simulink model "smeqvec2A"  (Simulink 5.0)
settings: Solver=ode45  StartTime=0.0  StopTime=3  MaxStep=1e-3  RelTol=1e-4  AbsTol=1e-4
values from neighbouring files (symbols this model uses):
  Bm = 0.10    (= 0.1)    [IMabc2.m]    (also in imabcparam.m = 0.01; IMabcrun0.m = 0.01; IMabcrun1.m = 0.001; IMcur0.m = 1e-06)
  H = 0.60    (= 0.6)    [IMabc2.m]    (also in IMcur0.m = 0.3; imdef0vec.m = 0.3; imdef1vec.m = 0.3; imdef2vec.m = 0.3)
  n0 = 0.98    [imdef0vec.m]    (also in imdef1vec.m = 0.978; imdef2vec.m; imdefrotflux.m; imdefSIvec1.m = 0.95)
  Te0 = 0.75/wo*p*(Is*conj(Is)*Req)    [imdefSIvec1.m]
  V = [Vas 0 0].'    [Actac.m]    (also in acttrcalc1.m = str2num(get(h,'string')); im3d.m = eval(get(hVs,'String')); IMabc2.m = [vas vbs vcs 0 0 0]'; IMabcf0.m = [vas vbs vcs 0 0 0]')
  wo = 2*pi*freq0    [calc0.m]    (also in IMabc2.m = 376.991118431; imabcparam.m = 376.991118431; IMabcrun0.m = 376.991118431; IMabcrun1.m = 376.991118431)
undefined symbols (not defined in the file or in its folder): delta0, fk0, L_1, ph, phif0, Rf, Rkd, Rkq, vf0
libraries: simulink x1

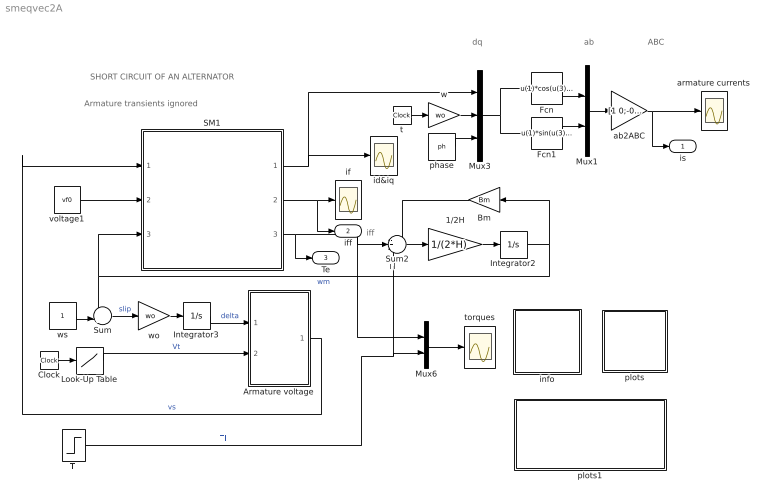
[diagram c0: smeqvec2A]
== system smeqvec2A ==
  note: Tl
  note: SHORT CIRCUIT OF AN ALTERNATOR
  note: iff
  note: Armature transients ignored
  note: ab
  note: ABC
  note: dq
  1/2H : Gain  Gain=1/(2*H)
  Armature voltage : Subsystem
  Bm : Gain  Orientation=left  Gain=Bm
  Clock : Clock
  Fcn : Fcn  Expr=u(1)*cos(u(3)+u(4))-u(2)*sin(u(3)+u(4))
  Fcn1 : Fcn  Expr=u(1)*sin(u(3)+u(4))+u(2)*cos(u(3)+u(4))
  Integrator2 : Integrator  InitialCondition=n0
  Integrator3 : Integrator  InitialCondition=delta0
  Look-Up Table : Lookup  InputValues=[0 0.1 0.1 5]  OutputValues=[V V 0 0]
  Mux1 : Mux  Inputs=2
  Mux3 : Mux  Inputs=3
  Mux6 : Mux  Inputs=2
  SM1 : Subsystem
  Sum : Sum  Inputs=-+|
  Sum2 : Sum  Inputs=-+-
  Tl : Step  Time=0  After=Te0  SampleTime=0
  ab2ABC : Gain  Gain=[1 0;-0.5 sqrt(3)/2;-0.5 -sqrt(3)/2]  Multiplication=Matrix(K*u)
  armature currents : Scope
  id&iq : Scope
  if : Scope
  info : Subsystem
  phase : Constant  Value=ph
  plots : Subsystem
  plots1 : Subsystem
  t : Clock
  torques : Scope
  voltage1 : Constant  Value=vf0
  w : Gain  Gain=wo
  wo : Gain  Gain=wo
  ws : Constant
  is : Outport
  iff : Outport  Port=2
  Te : Outport  Port=3
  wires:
  voltage1/1 -> SM1/2(vf)
  1/2H/1 -> Integrator2/1
  Sum2/1 -> 1/2H/1
  Bm/1 -> Sum2/1
  Mux6/1 -> torques/1
  ws/1 -> Sum/2
  Sum/1 -> wo/1  "slip"
  Armature voltage/1(vs) -> SM1/1(vs)  "vs"
  wo/1 -> Integrator3/1
  Integrator3/1 -> Armature voltage/1(delta)  "delta"
  Clock/1 -> Look-Up Table/1
  Look-Up Table/1 -> Armature voltage/2(Vt)  "Vt"
  Integrator2/1 -> Bm/1, Sum/1, SM1/3(wm)  "wm"
  Tl/1 -> Mux6/2, Sum2/3  "Tl"
  w/1 -> Mux3/2
  phase/1 -> Mux3/3
  t/1 -> w/1
  SM1/2(if) -> if/1, iff/1
  SM1/1(ia) -> id&iq/1, Mux3/1
  SM1/3(Te) -> Sum2/2, Mux6/1, Te/1
  Mux3/1 -> Fcn/1, Fcn1/1
  Fcn1/1 -> Mux1/2
  Fcn/1 -> Mux1/1
  Mux1/1 -> ab2ABC/1
  ab2ABC/1 -> armature currents/1, is/1

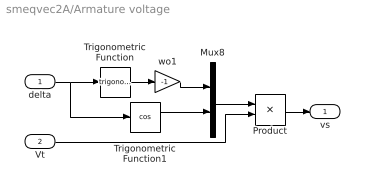
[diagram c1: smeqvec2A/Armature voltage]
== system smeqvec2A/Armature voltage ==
  delta : Inport
  Vt : Inport  Port=2
  Mux8 : Mux  Inputs=2
  Product : Product
  Trigonometric Function : Trigonometry
  Trigonometric Function1 : Trigonometry  Operator=cos
  wo1 : Gain  Gain=-1
  vs : Outport
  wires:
  delta/1 -> Trigonometric Function/1, Trigonometric Function1/1
  Trigonometric Function/1 -> wo1/1
  Mux8/1 -> Product/1
  wo1/1 -> Mux8/1
  Trigonometric Function1/1 -> Mux8/2
  Product/1 -> vs/1
  Vt/1 -> Product/2

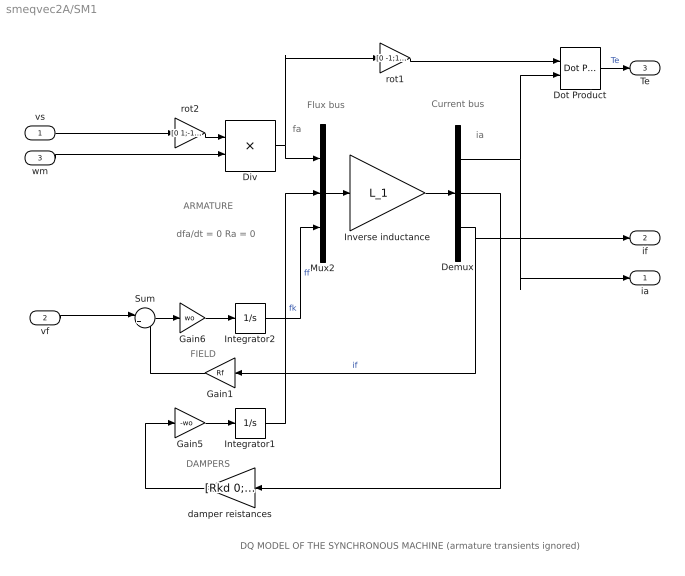
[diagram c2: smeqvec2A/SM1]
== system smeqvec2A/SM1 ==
  note: DAMPERS
  note: ARMATURE
  note: fa
  note: ia
  note: FIELD
  note: DQ MODEL OF THE SYNCHRONOUS MACHINE (armature transients ignored)
  note: Flux bus
  note: Current bus
  note: dfa/dt = 0 Ra = 0
  vs : Inport
  vf : Inport  Port=2
  wm : Inport  Port=3
  Demux : Demux  Outputs=3
  Div : Product  Inputs=*/  Multiplication=Matrix(*)
  Dot Product : simulink/Math Operations/Dot Product
  Gain1 : Gain  Orientation=left  Gain=Rf
  Gain5 : Gain  Gain=-wo
  Gain6 : Gain  Gain=wo
  Integrator1 : Integrator  InitialCondition=fk0
  Integrator2 : Integrator  InitialCondition=phif0
  Inverse inductance : Gain  Gain=L_1  Multiplication=Matrix(K*u)
  Mux2 : Mux  Inputs=3
  Sum : Sum  Inputs=|+-
  damper reistances : Gain  Orientation=left  Gain=[Rkd 0;0 Rkq]  Multiplication=Matrix(K*u)
  rot1 : Gain  Gain=[0 -1;1 0]  Multiplication=Matrix(K*u)
  rot2 : Gain  Gain=[0 1;-1 0]  Multiplication=Matrix(K*u)
  ia : Outport
  if : Outport  Port=2
  Te : Outport  Port=3
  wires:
  Gain5/1 -> Integrator1/1
  damper reistances/1 -> Gain5/1
  vs/1 -> rot2/1
  Gain6/1 -> Integrator2/1
  Sum/1 -> Gain6/1
  vf/1 -> Sum/1
  Gain1/1 -> Sum/2
  rot1/1 -> Dot Product/1
  Demux/1 -> Dot Product/2, ia/1
  Dot Product/1 -> Te/1  "Te"
  Mux2/1 -> Inverse inductance/1
  Inverse inductance/1 -> Demux/1
  Integrator1/1 -> Mux2/2  "fk"
  Integrator2/1 -> Mux2/3  "ff"
  Demux/2 -> damper reistances/1
  Demux/3 -> if/1, Gain1/1  "if"
  Div/1 -> Mux2/1, rot1/1
  rot2/1 -> Div/1
  wm/1 -> Div/2

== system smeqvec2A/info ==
  note: Synchronous machine transients under shortcircuit
  note: This demonstration illustrates the dynamics of a synchronous generator, initially at no load, following a three-phase short circuit at the terminals. The electric dynamic model of the synchronous machine is represented by a 3rd- order system accounting for the field and damper circuits but ignoring armature transients (dfa/dt = 0).

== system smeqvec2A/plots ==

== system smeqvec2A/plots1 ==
